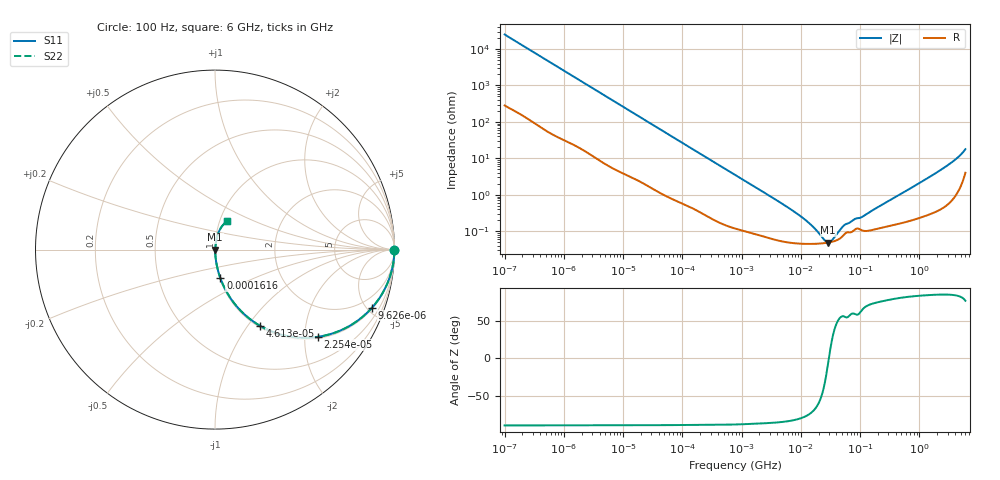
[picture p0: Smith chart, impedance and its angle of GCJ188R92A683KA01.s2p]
!Murata Part Number: GCJ188R92A683KA01
!These Parameters are Measured in Series Mode Connection
!Data Generated on Mar 13, 2026
!  o--ll--o
!Port1  Port2
!  o------o
!Operation Temp=25[degC], DC Bias Voltage=0[V]
!Freq. Start=100[Hz] Stop=6[GHz] 401[Steps]
# Hz S RI R 50
!Freq.(Hz) S11(Real) S11(Imag) S21(Real) S21(Imag) S12(Real) S12(Imag) S22(Real) S22(Imag)
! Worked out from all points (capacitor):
!   401 points, 100 Hz to 6 GHz, reference 50 ohm
!   read as one part in series: C = 63.4 nF near 109 Hz
!   lowest |Z| = 49.3 mohm at 29.12 MHz (marker M1)
!   series resonance near 29.73 MHz, so ESL is about 450 pH
!   S11 on the Smith chart (normalised r, x): 100 Hz: open; 9.626 kHz: 1.08, -5.39; 22.54 kHz: 1.04, -2.32; 46.13 kHz: 1.02, -1.14; 161.6 kHz: 1.01, -0.33; 6 GHz: 1.08, +0.35
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100  0.9999 -0.004  6.11e-05 0.004  6.11e-05 0.004  0.9999 -0.004
2008  0.9928 -0.0778  0.00718 0.0778  0.00718 0.0778  0.9928 -0.0778
5143  0.9595 -0.1906  0.0405 0.1906  0.0405 0.1906  0.9595 -0.1906
9626  0.8753 -0.323  0.1247 0.323  0.1247 0.323  0.8753 -0.323
14402  0.7622 -0.4177  0.2378 0.4177  0.2378 0.4177  0.7622 -0.4177
22537  0.5731 -0.4861  0.4269 0.4861  0.4269 0.4861  0.5731 -0.4861
40335  0.3022 -0.4504  0.6978 0.4504  0.6978 0.4504  0.3022 -0.4504
46134  0.2503 -0.4242  0.7497 0.4242  0.7497 0.4242  0.2503 -0.4242
78952  0.1063 -0.2982  0.8937 0.2982  0.8937 0.2982  0.1063 -0.2982
161617  0.0304 -0.1601  0.9696 0.1601  0.9696 0.1601  0.0304 -0.1601
774597  0.00243 -0.0351  0.9976 0.0351  0.9976 0.0351  0.00243 -0.0351
6353432  0.000507 -0.00426  0.9995 0.00426  0.9995 0.00426  0.000507 -0.00426
1.555665e7  0.000453 -0.00133  0.9995 0.00133  0.9995 0.00133  0.000453 -0.00133
2.545746e7  0.000476 -0.0003  0.9995 0.0003  0.9995 0.0003  0.000476 -0.0003
2.911731e7  0.000491 -4e-05  0.9995 4e-05  0.9995 4e-05  0.000491 -4e-05
3.330331e7  0.000513 0.000221  0.9995 -0.000221  0.9995 -0.000221  0.000513 0.000221
5.699437e7  0.000893 0.00128  0.9991 -0.00128  0.9991 -0.00128  0.000893 0.00128
8.154455e7  0.00111 0.00187  0.9989 -0.00187  0.9989 -0.00187  0.00111 0.00187
1.115611e8  0.00105 0.00233  0.999 -0.00233  0.999 -0.00233  0.00105 0.00233
3.124326e8  0.00145 0.0068  0.9985 -0.0068  0.9985 -0.0068  0.00145 0.0068
2.450438e9  0.00684 0.0508  0.9932 -0.0508  0.9932 -0.0508  0.00684 0.0508
6e9  0.065 0.1567  0.935 -0.1567  0.935 -0.1567  0.065 0.1567
